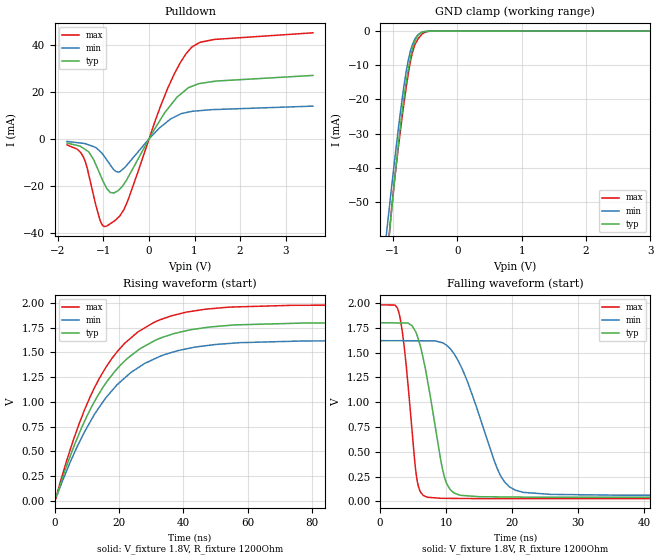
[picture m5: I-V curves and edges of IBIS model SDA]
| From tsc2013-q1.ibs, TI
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|   1.8V SDA Model
[Model] SDA
Model_type I/O_open_drain
Polarity   Non-Inverting
Enable   Active-Low
Vinl = 0.54
Vinh = 1.26
Vmeas = 0.9
Vref = 0.9
Cref = 15pF
Rref = 1200
|   typ   min   max
|   (nom PVT)   (Fast PVT)   (Slow PVT)
|   C_comp high output
C_comp   8.70246E-12   8.46524E-12   9.15466E-12
|   C_comp low output
|C_comp   9.45451E-12   9.41111E-12   9.49822E-12
|Where nom PVT is NOM Process, 1.8V,27C
|   Fast PVT is Strong Process, 2.07V, -40C
|   Slow PVT is Weak Process, 1.53V, 85C
[Voltage Range]   1.8   1.62   1.98
[Temperature Range]   30   88   -40
[Pullup Reference]   1.8   1.62   1.98
[Pulldown Reference]   0   0   0
[Power Clamp Reference]   1.8   1.62   1.98
[GND Clamp Reference]   0   0   0
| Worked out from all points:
|   slope of the pulldown table from 0 to 0.27 V, typ, clamps not added: 30.6 ohm
|   GND clamp passes 1 mA (typ) near -0.59 V on its own axis
|   falling waveform, V_fixture 1.8V, R_fixture 1200Ohm: 20-80 % time 2.74ns typ, 4.9ns min, 1.63ns max; typ from 1.8 V to 0.041 V
|   rising waveform, V_fixture 1.8V, R_fixture 1200Ohm: 20-80 % time 18.8ns typ, 19.6ns min, 17.8ns max; typ from 0.041 V to 1.8 V
[Pulldown]
|   Voltage   I(typ)   I(min)   I(max)
-1.8V     -1.785mA   -1.085mA   -2.549mA
-1.442V   -3.984mA   -1.903mA   -7.635mA
-1.322V   -5.598mA   -2.577mA   -15.41mA
-1.086V   -14.63mA   -5.118mA   -33.97mA
-932.3mV  -20.95mA   -8.825mA   -37.11mA
-721.2mV  -22.48mA   -13.92mA   -34.25mA
-549.6mV  -19.16mA   -12.44mA   -30.04mA
405.3mV   12.62mA    7.398mA    21.3mA
684.2mV   18.86mA    10.51mA    32.35mA
932.8mV   22.3mA     11.67mA    38.93mA
1.439V    24.51mA    12.49mA    42.32mA
3.6V      27mA       13.94mA    45.13mA
[GND Clamp]
|   Voltage   I(typ)   I(min)   I(max)
-1.8V     -218.2mA   -187.6mA   -259.9mA
-1.099V   -68.16mA   -59.13mA   -69.36mA
-1.059V   -60.12mA   -52.21mA   -60mA
-1.036V   -55.66mA   -48.37mA   -55.34mA
-977.4mV  -44.36mA   -38.55mA   -44.1mA
-908.8mV  -32.09mA   -27.59mA   -33.05mA
-787.1mV  -14.23mA   -11.17mA   -15.7mA
-700mV    -5.583mA   -4.146mA   -6.524mA
-640.8mV  -2.223mA   -1.844mA   -3.389mA
-569.8mV  -683.8uA   -517.8uA   -1.404mA
-419.2mV  -19.85uA   -21.03uA   -28.06uA
3.6V      0A         0A         0A
[POWER Clamp]
|   SCR cell for ESD function. Effects occurr above VDD x 2
|   Voltage   I(typ)   I(min)   I(max)
-1.8V     0A         0A         0A
0V        0A         0A         0A
3.6V      0A         0A         0A
[Ramp]
R_load = 1200
|   typ   min   max
dV/dt_r   1.05525/1.87695e-008  0.936119/1.95587e-008   1.17132/1.78529e-008
dV/dt_f   1.05526/2.73559e-009  0.936133/4.88116e-009   1.17132/1.62539e-009
[Falling Waveform]
V_fixture = 1.8V
V_fixture_min = 1.62V
V_fixture_max = 1.98V
R_fixture = 1200Ohm
|   Time   V(typ)   V(min)   V(max)
0s        1.8V       1.62V      1.98V
2.907ns   1.799V     1.619V     1.89V
3.935ns   1.798V     1.619V     1.389V
5.54ns    1.686V     1.619V     243.2mV
7.134ns   1.237V     1.619V     43.1mV
9.424ns   335.9mV    1.599V     31.43mV
10.61ns   119.8mV    1.54V      30.83mV
18.14ns   45.77mV    271.6mV    28.26mV
21.61ns   43.61mV    92.48mV    28.25mV
122.2ns   41.17mV    59.69mV    27.76mV
[Rising Waveform]
V_fixture = 1.8V
V_fixture_min = 1.62V
V_fixture_max = 1.98V
R_fixture = 1200Ohm
|   Time   V(typ)   V(min)   V(max)
0s        41.17mV    59.69mV    27.76mV
361.4ps   39.9mV     60.96mV    21.46mV
811.9ps   71.99mV    62.54mV    83.8mV
7.609ns   681.8mV    590.4mV    782.6mV
13.92ns   1.091V     949.8mV    1.242V
21.38ns   1.402V     1.232V     1.58V
30.47ns   1.608V     1.427V     1.797V
41.03ns   1.72V      1.536V     1.908V
55.76ns   1.777V     1.594V     1.959V
122.2ns   1.8V       1.62V      1.98V
